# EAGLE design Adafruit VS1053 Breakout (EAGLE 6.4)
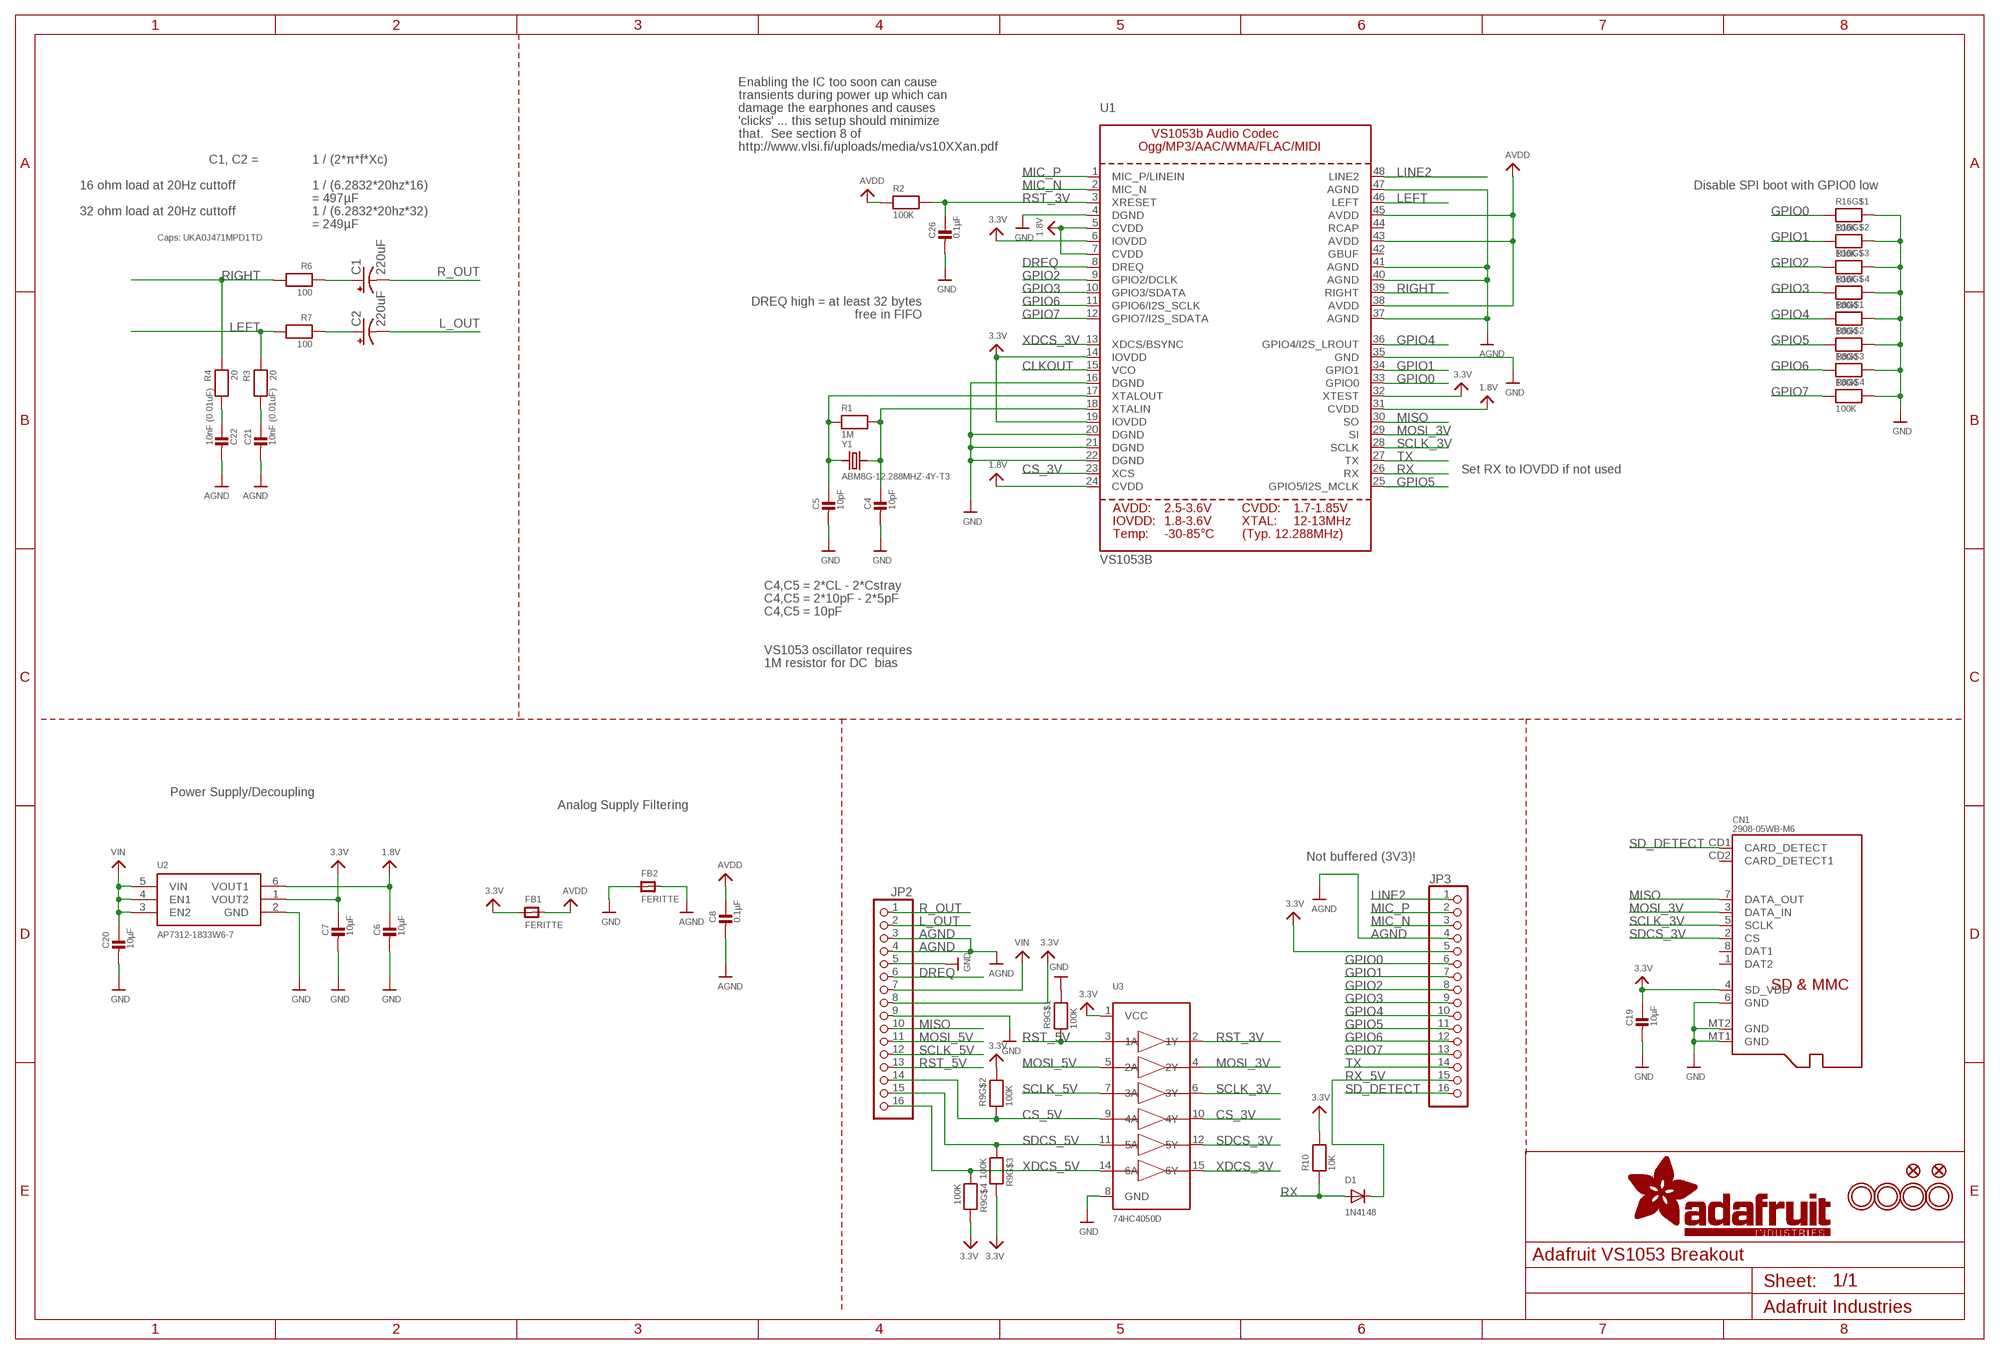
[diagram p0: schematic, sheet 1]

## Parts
C1  220uF  CPOL-USC  [PANASONIC_C]
C2  220uF  CPOL-USC  [PANASONIC_C]
C4  10pF  CAP_CERAMIC_0805MP  [_0805MP]
C5  10pF  CAP_CERAMIC_0805MP  [_0805MP]
C6  10µF  CAP_CERAMIC_0805MP  [_0805MP]
C7  10µF  CAP_CERAMIC_0805MP  [_0805MP]
C8  0.1µF  CAP_CERAMIC_0805MP  [_0805MP]
C19  10µF  CAP_CERAMIC_0805MP  [_0805MP]
C20  10µF  CAP_CERAMIC_0805MP  [_0805MP]
C21  10nF (0.01uF)  CAP_CERAMIC_0805MP  [_0805MP]
C22  10nF (0.01uF)  CAP_CERAMIC_0805MP  [_0805MP]
C26  0.1µF  CAP_CERAMIC_0805MP  [_0805MP]
CN1  2908-05WB-M6  MICROSD  [MICROSD]
D1  1N4148  DIODESOD-323  [SOD-323]
FB1  FERITTE  FERRITE_0805MP  [_0805MP]
FB2  FERITTE  FERRITE_0805MP  [_0805MP]
FID1  FIDUCIAL""  [FIDUCIAL_1MM]
FID2  FIDUCIAL""  [FIDUCIAL_1MM]
JP2  HEADER-1X16ROUND  [1X16_ROUND]
JP3  HEADER-1X16ROUND  [1X16_ROUND]
R1  1M  RESISTOR_0805MP  [_0805MP]
R2  100K  RESISTOR_0805MP  [_0805MP]
R3  20  RESISTOR_0805MP  [_0805MP]
R4  20  RESISTOR_0805MP  [_0805MP]
R6  100  RESISTOR_0805MP  [_0805MP]
R7  100  RESISTOR_0805MP  [_0805MP]
R8  100K  RESISTOR_4PACK  [RESPACK_4X0603]
R9  100K  RESISTOR_4PACK  [RESPACK_4X0603]
R10  10K  RESISTOR0805_NOOUTLINE  [0805-NO]
R16  100K  RESISTOR_4PACK  [RESPACK_4X0603]
U1  VS1053B  [LQFP48]
U2  AP7312-1833W6-7  VREG_SOT23-6_DUALAP7312  [SOT23-6]
U3  74HC4050D  [SOIC16]
U$50  MOUNTINGHOLE3.0THIN  [MOUNTINGHOLE_3.0_PLATEDTHIN]
U$51  MOUNTINGHOLE3.0THIN  [MOUNTINGHOLE_3.0_PLATEDTHIN]
U$52  MOUNTINGHOLE3.0THIN  [MOUNTINGHOLE_3.0_PLATEDTHIN]
U$53  MOUNTINGHOLE3.0THIN  [MOUNTINGHOLE_3.0_PLATEDTHIN]
Y1  ABM8G-12.288MHZ-4Y-T3  CRYSTAL3.2X2.5  [CRYSTAL_3.2X2.5]

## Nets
1.8V: C6.1 U1.5(CVDD) U1.7(CVDD) U1.24(CVDD) U1.31(CVDD) U2.6(VOUT1)
3.3V: C7.1 C19.1 CN1.4(SD_VDD) FB1.1 JP2.8 JP3.5 R9.5 R9.6 R9.7 R10.2 U1.6(IOVDD) U1.14(IOVDD) U1.19(IOVDD) U1.32(XTEST) U2.1(VOUT2) U3.1(VCC)
AGND: C8.2 C21.2 C22.2 FB2.2 JP2.3 JP2.4 JP3.4 U1.37(AGND) U1.40(AGND) U1.41(AGND) U1.47(AGND)
AVDD: C8.1 FB1.2 R2.1 U1.38(AVDD) U1.43(AVDD) U1.45(AVDD)
CLKOUT: U1.15(VCO)
CS_3V: U1.23(XCS) U3.10(4Y)
CS_5V: JP2.14 R9.2 U3.9(4A)
DREQ: JP2.6 U1.8(DREQ)
GND: C4.2 C5.2 C6.2 C7.2 C19.2 C20.2 C26.2 CN1.6(GND) CN1.MT1(GND) CN1.MT2(GND) FB2.1 JP2.5 JP2.9 R8.5 R8.6 R8.7 R8.8 R9.8 R16.5 R16.6 R16.7 R16.8 U1.4(DGND) U1.16(DGND) U1.20(DGND) U1.21(DGND) U1.22(DGND) U1.35(GND) U2.2(GND) U3.8(GND)
GPIO0: JP3.6 R16.1 U1.33(GPIO0)
GPIO1: JP3.7 R16.2 U1.34(GPIO1)
GPIO2: JP3.8 R16.3 U1.9(GPIO2/DCLK)
GPIO3: JP3.9 R16.4 U1.10(GPIO3/SDATA)
GPIO4: JP3.10 R8.1 U1.36(GPIO4/I2S_LROUT)
GPIO5: JP3.11 R8.2 U1.25(GPIO5/I2S_MCLK)
GPIO6: JP3.12 R8.3 U1.11(GPIO6/I2S_SCLK)
GPIO7: JP3.13 R8.4 U1.12(GPIO7/I2S_SDATA)
L_OUT: C2.- JP2.2
LEFT: R3.1 R7.2 U1.46(LEFT)
LEFT_FILTERED: C2.+ R7.1
LINE2: JP3.1 U1.48(LINE2)
MIC_N: JP3.3 U1.2(MIC_N)
MIC_P: JP3.2 U1.1(MIC_P/LINEIN)
MISO: CN1.7(DATA_OUT) JP2.10 U1.30(SO)
MOSI_3V: CN1.3(DATA_IN) U1.29(SI) U3.4(2Y)
MOSI_5V: JP2.11 U3.5(2A)
N$1: C5.1 R1.1 U1.17(XTALOUT) Y1.1
N$2: C4.1 R1.2 U1.18(XTALIN) Y1.2
N$5: C21.1 R3.2
N$6: C22.1 R4.2
R_OUT: C1.- JP2.1
RIGHT: R4.1 R6.2 U1.39(RIGHT)
RIGHT_FILTERED: C1.+ R6.1
RST_3V: C26.1 R2.2 U1.3(XRESET) U3.2(1Y)
RST_5V: JP2.13 R9.1 U3.3(1A)
RX: D1.A R10.1 U1.26(RX)
RX_5V: D1.C JP3.15
SCLK_3V: CN1.5(SCLK) U1.28(SCLK) U3.6(3Y)
SCLK_5V: JP2.12 U3.7(3A)
SD_DETECT: CN1.CD1(CARD_DETECT) JP3.16
SDCS_3V: CN1.2(CS) U3.12(5Y)
SDCS_5V: JP2.15 R9.3 U3.11(5A)
TX: JP3.14 U1.27(TX)
VIN: C20.1 JP2.7 U2.3(EN2) U2.4(EN1) U2.5(VIN)
XDCS_3V: U1.13(XDCS/BSYNC) U3.15(6Y)
XDCS_5V: JP2.16 R9.4 U3.14(6A)
Unconnected: CN1.1(DAT2) CN1.8(DAT1) CN1.CD2(CARD_DETECT1) U1.42(GBUF) U1.44(RCAP)

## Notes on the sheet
- Enabling the IC too soon can cause
- transients during power up which can
- damage the earphones and causes
- 'clicks' ... this setup should minimize
- that.  See section 8 of
- http://www.vlsi.fi/uploads/media/vs10XXan.pdf
- C1, C2 = | 1 / (2*π*f*Xc)
- 16 ohm load at 20Hz cuttoff | 1 / (6.2832*20hz*16) | Disable SPI boot with GPIO0 low
- = 497µF
- 32 ohm load at 20Hz cuttoff | 1 / (6.2832*20hz*32)
- = 249µF
- Caps: UKA0J471MPD1TD
- DREQ high = at least 32 bytes
- free in FIFO
- Set RX to IOVDD if not used
- C4,C5 = 2*CL - 2*Cstray
- C4,C5 = 2*10pF - 2*5pF
- C4,C5 = 10pF
- VS1053 oscillator requires
- 1M resistor for DC  bias
- Power Supply/Decoupling
- Analog Supply Filtering
- Not buffered (3V3)!

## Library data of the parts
C1 C2 = rcl:CPOL-US: POLARIZED CAPACITOR, American symbol
C4-C8 C19-C22 C26 = microbuilder:CAP_CERAMIC: Ceramic Capacitors
CN1 = microbuilder:MICROSD: MicroSD/Transflash Card Holder with SPI pinout 3M: 2908-05WB-MG 4UConnector: 19656 Footprint courtesy: Adafruit Industries
D1 = microbuilder:DIODE: Diode
FB1 FB2 = microbuilder:FERRITE: Ferrite Bead
FID1 FID2 = microbuilder:FIDUCIAL: Fiducial Alignment Points; BOM: EXCLUDE
JP2 JP3 = microbuilder:HEADER-1X16: PIN HEADER
R1-R4 R6 R7 R10 = microbuilder:RESISTOR: Resistors
R8 R9 R16 = microbuilder:RESISTOR_4PACK: Resistor Packs (4 resistors) 4 x 0603 10K 1/16W - Digikey: YC164J-10KCT-ND
U1 = microbuilder:VS1053B: VS1053b Audio Codec - Ogg Vorbis/MP3/AAC/WMA/FLAC/MIDI
U2 = microbuilder:VREG_SOT23-6_DUAL: Dual Output SOT23-6 Linear Regulators Diodes Inc. AP7312 - Dual 150mA LDO Linear Regulator 0.2V dropout, 150mA output, 2-6V Input AP7312-1833W6-7 - 1.8V/3.3V SOT23-6 (Digikey: AP7312-1833W6-7DICT-ND) MIC5320 - Dual 150mA ULDO Linear Regulator Ultra-low 35mV dropout at 150mA, 2.3-5.5V Input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
U3 = microbuilder:74HC4050D: 6-channel level shifter 74HC4050D - 2V-6V Supply SOIC16 Digikey: 74HC4050D,653-ND Mouser: 771-74HC4050D-T TSSOP16 Digikey: 296-9215-1-ND Mouser:
U$50-U$53 = microbuilder:MOUNTINGHOLE: Mounting Hole; BOM: EXCLUDE
Y1 = microbuilder:CRYSTAL: Crystals

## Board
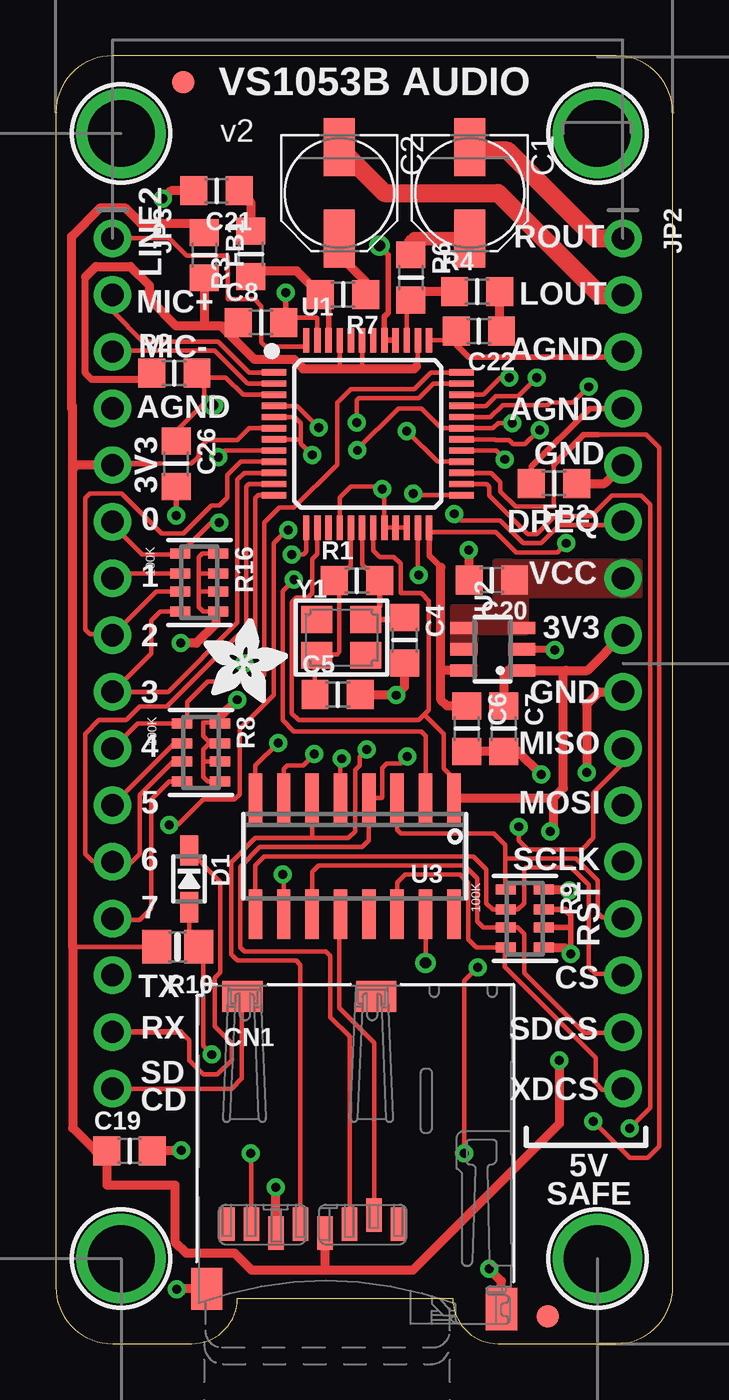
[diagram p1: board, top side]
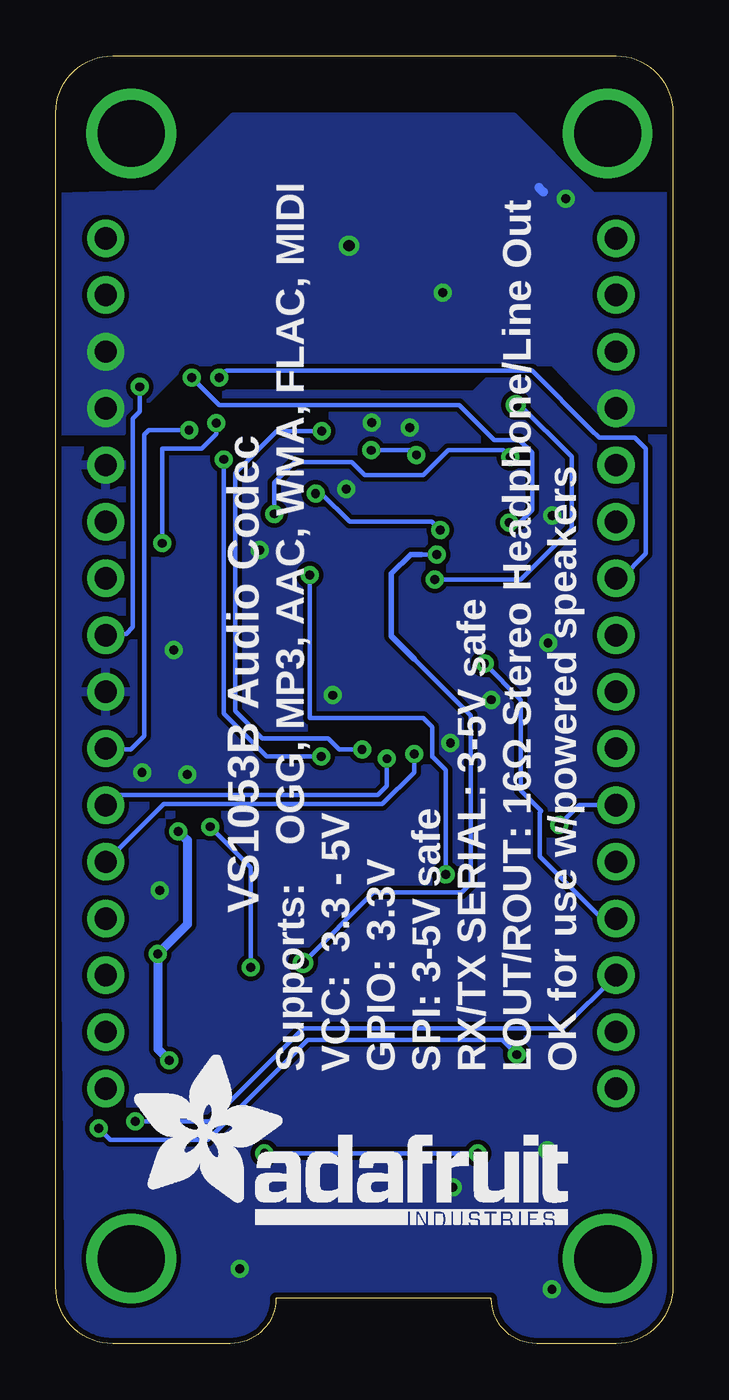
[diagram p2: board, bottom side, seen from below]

Size 27.64 x 57.71 mm. Coordinates in mm from the lower left corner, seen from the top.
Outline: 19.81,0 25.09,0 arc90 27.64,2.54 27.64,55.17 arc90 25.09,57.71 2.54,57.71 arc90 0,55.17 0,2.54 arc90 2.54,0 6.1,0 arc90 8.13,2.03 17.78,2.03 arc90 19.81,0
Copper layers (1*16): Top 0.035mm / dielectric 1.5mm / Bottom 0.035mm
Design rules "adafruit *": minimum track width 8mil, minimum drill 15.5mil, track to track 8mil, track to pad 8mil, pad to pad 8mil, via to via 8mil, smd to smd 8mil, copper to edge 10mil, drill to drill 8mil, minimum pad ring 10mil, minimum via ring 8mil, stop-mask expansion 4mil, vias tented up to drill 20mil, thermal gap 10mil

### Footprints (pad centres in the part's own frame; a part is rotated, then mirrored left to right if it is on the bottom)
PANASONIC_C = smd 2.6 x 1.4: + 2.05,0; - -2.05,0
_0805MP = smd 1.2 x 1.3: 1 -1.016,0; 2 1.016,0
MICROSD = smd 0.7 x 1.5: 1 9,-10.64; 2 7.9,-10.24; 3 6.8,-10.64; 4 5.7,-11.04; 5 4.6,-10.64; 6 3.5,-11.04; 7 2.4,-10.64; 8 1.3,-10.64 | smd 1.8 x 1.4: CD1 2,-0.44; CD2 8,-0.44 | smd 1.4 x 1.9: MT1 0.4,-13.54; MT2 13.6,-14.44
SOD-323 = smd 1.35 x 0.8: A 1.27,0; C -1.27,0
FIDUCIAL_1MM = smd 1 x 1: 1 0,0
1X16_ROUND = drill 1 pad 1.676: 1 -19.05,0; 2 -16.51,0; 3 -13.97,0; 4 -11.43,0; 5 -8.89,0; 6 -6.35,0; 7 -3.81,0; 8 -1.27,0; 9 1.27,0; 10 3.81,0; 11 6.35,0; 12 8.89,0; 13 11.43,0; 14 13.97,0; 15 16.51,0; 16 19.05,0
RESPACK_4X0603 = smd 0.45 x 0.9: 1 -1.3,-0.85; 2 -0.4,-0.85; 3 0.4,-0.85; 4 1.3,-0.85; 5 1.3,0.85; 6 0.4,0.85; 7 -0.4,0.85; 8 -1.3,0.85
0805-NO = smd 1.3 x 1.5: 1 -0.95,0; 2 0.95,0
LQFP48 = smd 1.1 x 0.285: 1 -4.2,2.75; 2 -4.2,2.25; 3 -4.2,1.75; 4 -4.2,1.25; 5 -4.2,0.75; 6 -4.2,0.25; 7 -4.2,-0.25; 8 -4.2,-0.75; 9 -4.2,-1.25; 10 -4.2,-1.75; 11 -4.2,-2.25; 12 -4.2,-2.75; 25 4.2,-2.75; 26 4.2,-2.25; 27 4.2,-1.75; 28 4.2,-1.25; 29 4.2,-0.75; 30 4.2,-0.25; 31 4.2,0.25; 32 4.2,0.75; 33 4.2,1.25; 34 4.2,1.75; 35 4.2,2.25; 36 4.2,2.75 | smd 0.285 x 1.1: 13 -2.75,-4.2; 14 -2.25,-4.2; 15 -1.75,-4.2; 16 -1.25,-4.2; 17 -0.75,-4.2; 18 -0.25,-4.2; 19 0.25,-4.2; 20 0.75,-4.2; 21 1.25,-4.2; 22 1.75,-4.2; 23 2.25,-4.2; 24 2.75,-4.2; 37 2.75,4.2; 38 2.25,4.2; 39 1.75,4.2; 40 1.25,4.2; 41 0.75,4.2; 42 0.25,4.2; 43 -0.25,4.2; 44 -0.75,4.2; 45 -1.25,4.2; 46 -1.75,4.2; 47 -2.25,4.2 | smd 0.28 x 1.1: 48 -2.75,4.2
SOT23-6 = smd 0.55 x 1.2: 1 -0.95,-1.3; 2 0,-1.3; 3 0.95,-1.3; 4 0.95,1.3; 5 0,1.3; 6 -0.95,1.3
SOIC16 = smd 0.6 x 2.2: 1 -4.445,-2.6; 2 -3.175,-2.6; 3 -1.905,-2.6; 4 -0.635,-2.6; 5 0.635,-2.6; 6 1.905,-2.6; 7 3.175,-2.6; 8 4.445,-2.6; 9 4.445,2.6; 10 3.175,2.6; 11 1.905,2.6; 12 0.635,2.6; 13 -0.635,2.6; 14 -1.905,2.6; 15 -3.175,2.6; 16 -4.445,2.6
MOUNTINGHOLE_3.0_PLATEDTHIN = drill 3 pad 3.6: P$1 0,0
CRYSTAL_3.2X2.5 = smd 1.4 x 1.2: 1 -1.1,-0.8; 2 1.1,0.8; GND1 -1.1,0.8; GND2 1.1,-0.8

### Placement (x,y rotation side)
C1  18.54,51.56 270 top
C2  12.7,51.56 270 top
C4  15.62,31.52 270 top
C5  12.62,29.08 0 top
C6  18.41,27.56 270 top
C7  20.07,27.56 270 top
C8  9.19,45.76 0 top
C19  3.3,8.64 0 top
C20  19.53,34.21 180 top
C21  7.2,51.66 180 top
C22  18.95,45.37 180 top
C26  5.38,39.43 270 top
CN1  6.36,16 0 top
D1  5.97,20.83 270 top
FB1  6.66,48.77 270 top
FB2  22.32,38.55 180 top
FID1  5.71,56.52 0 top
FID2  22.04,1.22 0 top
JP2  25.4,30.48 270 top
JP3  2.54,30.48 270 top
R1  13.49,34.19 0 top
R2  5.31,43.49 0 top
R3  8.73,48.83 90 top
R4  18.87,47.14 0 top
R6  15.91,47.77 270 top
R7  12.86,47.01 180 top
R8  6.5,26.49 270 top
R9  21.01,19.05 270 top
R10  5.46,17.78 180 top
R16  6.43,34.11 270 top
U1  13.97,40.77 0 top
U2  19.57,31.12 90 top
U3  13.39,21.84 180 top
U$31  [ADAFRUIT_3.5MM]  6.6,28.7 0 top
U$50  2.92,3.81 0 top
U$51  24.26,3.81 0 top
U$52  24.26,54.23 0 top
U$53  2.92,54.23 0 top
U$55  [ADAFRUIT_TEXT_20MM]  24.28,5.33 0 bottom
Y1  12.79,31.64 0 top

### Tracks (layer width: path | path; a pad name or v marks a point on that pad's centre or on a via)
1.8V  (via drill 0.4)
  Top 0.203: U1.5 10.71,41.52 10.97,41.25 10.97,40.54 | 10.97,40.54 10.97,40.34 v11.48,39.83 | U1.7 10.95,40.52 10.97,40.54 | v22.86,35.87 22.45,35.46 20.62,35.46 19.71,36.37 16.76,36.37 16.72,36.42 U1.24 | v13.51,40.03 13.46,40.03 15.34,41.91 16.38,41.91 17.27,41.02 U1.31 | v20.45,41.25 19.82,41.25 19.81,41.25 19.58,41.02 U1.31 | U1.31
  Top 0.254: U1.24 16.72,35.33 17.25,34.8
  Top 0.406: C6.1 17.53,28.57 17.25,28.85 17.25,30.23 | 17.25,30.23 17.25,34.8 | U2.6 17.3,30.17 17.25,30.23
  Bottom 0.203: v13.51,40.03 11.68,40.03 v11.48,39.83 | v22.86,35.87 22.86,40.1 21.1,40.1 20.45,40.75 v20.45,41.25
3.3V  (via drill 0.4)
  Top 0.203: 16.51,28.19 16.71,28.4 16.71,33.27 16.36,33.63 15.44,33.63 15.44,34.95 15.14,35.26 14.5,35.26 14.22,35.54 U1.19 | 16.51,28.19 16.26,27.94 10.87,27.94 10.57,28.25 10.57,33.22 10.77,33.43 11.28,33.43 11.48,33.63 11.48,35.15 11.72,35.39 U1.14 | U3.1 17.78,24.5 17.78,25.38 17.37,25.78 17.37,27.33 16.51,28.19 | v23.88,42.88 23.16,42.16 22.15,42.16 22.04,42.06 20.01,42.06 19.47,41.52 U1.32 | U1.6 8.66,41.02 8.13,40.49 6.79,40.49 6.4,40.1 6.4,39.76 | 6.4,39.76 6.4,39.7 | 4.42,39.43 6.07,39.43 6.4,39.76 | R10.2 0.75,17.78
  Top 0.254: R9.7 22.82,19.45 23.06,19.2 23.06,18.59 | 23.06,18.59 v23.06,17.48 | R9.6 23.01,18.65 23.06,18.59 | 4.42,39.43 2.6,39.43 JP3.5
  Top 0.406: 0.71,41.91 0.71,42.04 | 0.71,42.04 0.71,49.61 2,50.9 3.1,50.9 3.8,50.2 6.5,50.2 6.5,49.95 FB1.1 | C7.1 20.07,29.97 20.26,30.17 U2.1 22.86,30.17 | 22.86,30.17 23.82,30.17 JP2.8 | U3.1 22.29,24.44 | 22.29,24.44 22.73,24.89 22.73,30.04 22.86,30.17 | CN1.4 12.06,3.38 11.99,3.3 | R9.5 22.79,17.75 v23.06,17.48 | v22.55,12.7 22.55,9.86 16,3.3 11.99,3.3 | 11.99,3.3 8.76,3.3 8,4.06 5.84,4.06 5.33,4.57 5.33,7.11 2.29,7.11 C19.1 1.78,8.64 0.75,9.67 0.75,17.78 0.75,39.2 | 22.29,24.44 22.29,23.1 v22.15,22.96 | 0.75,39.2 0.75,42 0.71,42.04 | JP3.5 0.92,39.37 0.75,39.2
  Bottom 0.203: v23.88,42.88 23.88,41.76 24.18,41.45 24.18,32.11 24.49,31.8 25.35,31.8 JP2.8
  Bottom 0.406: v22.55,12.7 23.06,13.21 v23.06,17.48 21.74,18.8 21.74,22.55 v22.15,22.96
AGND  (via drill 0.4, 0.5)
  Top 0.203: U1.37 17.8,44.97 17.94,44.83 | U1.47 11.72,45.94 11.68,45.97 10.42,45.97 C8.2
  Top 0.254: FB2.2 21.3,39.3 23.91,41.91 JP2.4 | C22.2 17.94,44.83 17.94,44.76 18.5,44.2 25.15,44.2 JP2.3 | U1.40 U1.41 14.72,46.02 14.9,46.2 14.9,48.8 v14.5,49.2 | 10.3,45.85 v10.3,47.1 | 10.64,46.2 10.56,46.12 | 10.56,46.12 10.3,45.85 | 10.54,46.12 10.56,46.12 | 10.3,45.85 C8.2
  Top 0.406: C21.2 5.16,51.66 v4.8,51.3
  Bottom 0.254: v14.5,49.2 14.6,49.2 14.7,49.3
  Bottom 0.406: 6,51.8 5.8,51.6
  pour Bottom (no thermals): 0,41.18 2.77,41.18 5.38,43.89 21.84,43.89 24.59,41.15 24.59,40.8 26.11,40.8 27.61,40.78 27.61,51.49 23.16,51.61 19.71,55.07 7.11,55.07 3.56,51.51 0,51.51
AVDD
  Top 0.203: U1.38 16.22,43.85 16.15,43.79 | 13.82,43.69 13.72,43.79 U1.43 | U1.45 12.72,43.71 12.7,43.69 | 3.71,43.2 4.09,43.59 | 8.01,45.6 8.18,45.6 C8.1
  Top 0.254: 4.09,43.59 4.19,43.59 R2.1 | 7.71,45.6 8.01,45.6
  Top 0.305: 3.71,43.2 1.6,43.2 1.32,43.48 1.32,47.79
  Top 0.406: 16.15,43.79 16.05,43.69 13.82,43.69 12.7,43.69 11.07,43.69 10.66,44.1 8.9,44.1 7.4,45.6 | 1.32,47.79 1.79,48.26 3.34,48.26 4.2,47.4 4.2,46.8 5.4,45.6 6.7,45.6 | 7.4,45.6 6.7,45.6 | 7.4,45.6 7.71,45.6 | FB1.2 6.66,45.64 6.7,45.6
CS_3V  (via drill 0.4)
  Top 0.203: U3.10 10.21,20.98 v10.16,21.03 | U1.23 16.22,34.48 v16.26,34.44
  Bottom 0.203: v10.16,21.03 10.16,25.7 10.74,26.29 10.77,26.29 10.77,27.64 11.18,28.04 16.26,28.04 v16.26,34.44
CS_5V
  Top 0.203: U3.9 8.94,21.44 9.35,21.84 18.69,21.84 19.28,21.26 19.28,19.74 19.56,19.45 R9.2 20.7,19.45 20.98,19.74 20.98,21.26 21.06,21.34 23.09,21.34 23.88,20.55 23.88,16.87 24.18,16.56 25.35,16.56 JP2.14
DREQ  (via drill 0.4)
  Top 0.203: 25.35,36.88 JP2.6 25.25,36.68 22.55,36.68 21.74,35.87 20.93,35.87 19.91,36.88 18.16,36.88 v17.86,37.19 | U1.8 7.58,40.02 v7.29,39.73
  Bottom 0.203: v7.29,39.73 7.59,40.03 10.06,40.03 11.18,38.91 13.79,38.91 14.38,39.5 16.94,39.5 17.86,38.58 v17.86,37.19 17.88,37.19
GND  (via drill 0.4)
  Top 0.203: R8.5 6.81,25.19 6.6,25.4 6.6,26.11 | 6.6,26.11 6.6,26.62 6.88,26.89 R8.7 6.94,26.89 6.6,27.23 6.6,27.84 7.31,27.84 R8.8 | R8.6 6.62,26.09 6.6,26.11 | R16.8 6.56,35.41 6.4,35.26 6.4,34.54 | 6.4,34.54 6.4,33.73 | 6.4,33.73 6.4,33.02 6.6,32.82 7.17,32.82 | R16.6 6.42,33.71 6.4,33.73 | R16.7 6.43,34.51 6.4,34.54 | U1.16 12.72,37.92 13.21,38.41 14.53,38.41 v14.63,38.3 14.72,38.21 U1.20 U1.21 U1.22 | U1.35 16.91,43.02 16.26,42.37 13.56,42.37 13.49,42.29 v13.49,41.27 | U1.4 10.81,42.02 v11.79,41.05 | U3.8 8.94,25.91 v9.96,26.92 | 7.37,28.1 7.38,28.09
  Top 0.254: C26.2 5.38,37.12 v5.4,37.1
  Top 0.305: U2.2 22.32,31.12 v22.35,31.09
  Top 0.406: v8.13,28.85 7.37,28.1 7.37,27.81 R8.8 | v5.59,31.39 6.3,31.39 7.18,32.27 7.18,32.71 R16.5 7.18,32.81 7.17,32.82 | C20.2 18.52,35.53 v18.49,35.56 | v23.77,25.6 23.77,28.65 24.33,29.21 JP2.9 | C6.2 C7.2 20.7,26.54 v21.74,25.5 | C5.2 15.21,29.08 v15.24,29.06 15.62,29.44 C4.2 | R9.8 22.96,20.35 v22.99,20.32 | CN1.6 v9.86,7.01 | CN1.MT1 5.43,2.46 v5.41,2.44 | CN1.MT2 19.96,2.8 v19.41,3.35 | v5.61,8.66 5.59,8.64 C19.2 | FB2.1 24.58,38.55 JP2.5
  pour Bottom: 0,40.57 2.77,40.47 5.8,43.2 8.1,43.3 8.9,42.5 21.54,42.57 23.27,40.84 23.27,39.99 27.43,39.99 27.03,0 0,0
GPIO0  (via drill 0.4)
  Top 0.203: JP3.6 2.54,36.68 3.86,35.36 5.62,35.36 5.62,35.37 R16.1 6.95,36.79 7.05,36.79 | v21.54,43.28 20.72,42.47 19.71,42.47 19.26,42.02 U1.33
  Top 0.254: 7.05,36.79 v7.32,36.79
  Bottom 0.203: v21.54,43.28 20.32,42.06 9.56,42.06 8,40.5 6.87,40.5 6.3,39.93 6.3,37.35 6.86,36.79
  Bottom 0.254: 6.86,36.79 | 6.86,36.79 v7.32,36.79
GPIO1  (via drill 0.4)
  Top 0.203: 2.56,34.31 JP3.7 2.76,34.51 R16.2 | U1.34 19.15,42.52 19.91,43.28 v20.32,43.28
  Bottom 0.203: 20.22,43.18 v20.32,43.28 20,43.6 6.3,43.6 3.66,40.96 3.3,40.6 1.7,40.6 1.2,40.1 1.2,35.4 2.31,34.29 JP3.7
GPIO2
  Top 0.203: R16.3 4.5,33.71 JP3.8 2.49,31.8 1.52,31.8 1.32,32 1.32,37.9 1.52,38.1 2.95,38.1 4.75,36.3 5.7,36.3 6.96,37.55 7.32,37.55 7.67,37.91 7.67,38.91 8.28,39.52 U1.9
GPIO3
  Top 0.203: U1.10 8.44,39.02 8.13,38.71 8.13,32.31 5.03,29.21 JP3.9 4.27,30.94 4.27,32.41 4.67,32.81 R16.4
  Bottom 0.203: 2.59,29.16 JP3.9
GPIO4
  Top 0.203: JP3.10 3.66,27.79 R8.1 5.89,28.03 5.89,28.75 6.81,29.67 9.04,29.67 9.35,29.97 9.35,36.8 10.01,37.47 10.67,37.47 12.6,39.4 12.6,42.16 13.21,42.77 16.05,42.77 16.8,43.52 U1.36
GPIO5  (via drill 0.4)
  Top 0.203: R8.2 5.3,26.89 JP3.11 | v5.08,23.24 5.46,23.24 6.6,24.38 8,24.38 8.23,24.61 8.23,27.53 9.75,29.06 9.75,35.87 10.34,36.45 v10.41,36.45 | v16,38.1 16.09,38.02 U1.25
  Bottom 0.203: JP3.11 4.19,24.13 v5.08,23.24 | v10.41,36.45 10.79,36.83 14.48,36.83 15.75,38.1 v16,38.1
GPIO6
  Top 0.203: R8.3 5.26,26.09 3.76,24.59 3.76,21.95 3.35,21.54 2.59,21.54 JP3.12 2.49,21.64 1.63,21.64 1.32,21.95 1.32,27.33 1.93,27.94 3.15,27.94 3.76,28.55 4.98,28.55 8.53,32.11 8.53,38.41 8.65,38.52 U1.11
GPIO7  (via drill 0.4)
  Top 0.203: JP3.13 2.59,19 3.76,19 4.27,19.51 4.27,24.38 5.08,25.19 R8.4 | U1.12 9.06,38.02 8.94,37.9 8.94,30.99 v8.43,30.48
  Bottom 0.203: v8.43,30.48 6.81,28.85 6.81,24.79 5.89,23.88 5.97,23.8 5.97,21.84 3.17,19.05 JP3.13
L_OUT
  Top 0.813: C2.- 12.7,53.59 14.73,51.56 19.81,51.56 24.38,46.99 JP2.2
LEFT
  Top 0.254: U1.46 12.22,46.84 12.05,47.01 R7.2
  Top 0.406: R3.1 8.97,48.06 10.8,48.06 R7.2
LEFT_FILTERED
  Top 0.406: R7.1 13.88,47.59 12.7,48.77 C2.+
LINE2
  Top 0.203: JP3.1 5.07,49.53 5.85,48.75 7.65,48.75 7.7,48.7 7.7,46.8 8.9,46.8 9.2,46.5 9.2,44.87 9.4,44.67 11.22,44.67 U1.48
MIC_N
  Top 0.203: U1.2 8.6,43.02 7.12,44.5 2.6,44.5 arc60 JP3.3
MIC_P
  Top 0.203: U1.1 8.67,43.52 7.28,44.9 3.9,44.9 2.54,46.26 JP3.2
MISO  (via drill 0.4)
  Top 0.203: CN1.7 8.76,8.51 v8.74,8.53 | v18.29,8.53 18.29,16.26 v18.9,16.87 | v20.73,23.16 20.73,22.55 21.13,22.15 23.57,22.15 24.08,22.66 24.08,24.69 25.3,25.91 25.3,26.57 JP2.10 | U1.30 19.69,40.52 19.71,40.5 20.3,40.5 20.5,40.3 21,40.3 21.65,40.95 v21.67,40.95
  Bottom 0.203: JP2.10 25.35,26.62 24.28,26.62 23.67,27.23 23.67,40.74 23.47,40.95 v21.67,40.95 | v8.74,8.53 v18.29,8.53 | v18.9,16.87 18.9,21.34 v20.73,23.16
MOSI_3V  (via drill 0.4)
  Top 0.203: CN1.3 13.16,13.77 12.29,14.63 12.29,17.37 12.09,17.58 8.43,17.58 8.26,17.75 8.26,21.36 9.14,22.25 13.72,22.25 14.02,22.55 U3.4 14.59,24.44 14.63,24.49 14.63,25.81 14.83,26.01 15.44,26.01 v15.75,26.31 | v20.11,39.63 19.72,40.02 U1.29
  Bottom 0.203: v15.75,26.31 18.19,26.31 20.11,28.24 v20.11,39.63
MOSI_5V  (via drill 0.4)
  Top 0.203: U3.5 12.75,26.16 v12.8,26.21
  Bottom 0.203: v12.8,26.21 12.8,24.99 13.21,24.59 24.94,24.59 JP2.11
N$1
  Top 0.203: R1.1 12.24,34.19 | 11.63,29.1 C5.1 11.61,30.76 Y1.1 11.73,30.89 12.6,30.89 12.7,30.99 12.7,33.83 12.47,34.06 R1.1 | U1.17 13.22,34.86 12.55,34.19 R1.1
N$2
  Top 0.203: U1.18 13.72,34.92 14.45,34.19 R1.2
  Top 0.254: R1.2 14.5,33.06 Y1.2 15.62,32.44 C4.1
N$5
  Top 0.406: C21.1 8.73,51.14 R3.2
N$6
  Top 0.406: C22.1 19.89,45.37 R4.2
R_OUT
  Top 0.813: JP2.1 24.17,49.53 20.25,53.45 18.7,53.45 C1.-
RIGHT
  Top 0.203: 15.71,46.76 15.71,46.95 15.9,47.14 | U1.39 15.72,46.57 R6.2
  Top 0.254: 15.71,46.76 R6.2
  Top 0.406: R4.1 15.9,47.14 15.71,47.14
RIGHT_FILTERED
  Top 0.61: C1.+ 16.07,49.51 15.91,49.35 R6.1
RST_3V  (via drill 0.4, 0.5)
  Top 0.203: U1.3 8.38,42.52 7.62,43.28 6.53,43.28 R2.2 6.43,43.39 6.43,43.08 6.66,42.85 6.66,42.49 6.99,42.16 6.99,42.11 v7.04,42.06 6.56,42.06 5.38,40.88 C26.1 | U3.2 16.56,27.23 16.36,27.43 10.67,27.43 10.16,27.94 10.16,33.73 v10.67,34.24
  Bottom 0.203: v10.67,34.24 6.81,34.24 4.53,36.51 4.53,39.75 6.84,42.06 v7.04,42.06
RST_5V
  Top 0.203: U3.3 15.29,23.01 15.44,22.86 19.61,22.86 20.13,22.34 20.13,21.74 | 20.13,21.74 23.29,21.74 24.28,20.75 24.28,19.3 24.49,19.1 25.35,19.1 JP2.13 | 20.13,21.74 20.13,20.32 R9.1
RX  (via drill 0.4)
  Top 0.203: U1.26 19.29,38.52 19.41,38.4 19.41,37.99 21.13,36.27 21.54,36.27 22.35,37.08 23.98,37.08 24.89,38 26.21,38 26.62,37.59 26.62,10.57 v25.7,9.65 | v6.99,12.95 6.6,13.34 6.6,17.59 R10.1 5.97,18.22 D1.A
  Bottom 0.203: v25.7,9.65 25.2,9.14 20.83,9.14 16.36,13.61 7.64,13.61 v6.99,12.95
RX_5V
  Top 0.203: 5.59,13.97 5.97,13.59 5.97,12.7 6.6,12.06 7.24,12.06 7.87,12.7 7.87,13.46 7.11,14.22 7.11,16.38 7.37,16.64 7.37,20.7 D1.C
  Top 0.254: JP3.15 5.59,13.97
SCLK_3V  (via drill 0.4)
  Top 0.203: CN1.5 10.96,16.98 10.77,17.17 8.13,17.17 7.85,17.45 7.85,21.57 8.94,22.66 11.48,22.66 | 11.48,22.66 13.11,22.66 13.41,22.96 13.41,25.7 13.61,25.91 13.61,26.31 v13.92,26.62 | 11.48,22.66 U3.6 | U1.28 17.1,39.52 v15.72,40.89
  Bottom 0.203: v15.72,40.89 17.73,40.89 19.61,39.01 19.61,28.35 18.39,27.13 15.44,27.13 14.94,26.62 v13.92,26.62
SCLK_5V  (via drill 0.4)
  Top 0.203: U3.7 10.21,25.76 10.36,25.91 11.07,25.91 v11.58,26.42
  Bottom 0.203: v11.58,26.42 11.58,25.6 13.01,24.18 22.81,24.18 JP2.12
SD_DETECT
  Top 0.203: JP3.16 7.87,11.43 8.33,11.89 8.33,15.54 CN1.CD1
SDCS_3V
  Top 0.203: CN1.2 14.26,13.48 12.7,15.04 12.7,19.19 U3.12
SDCS_5V
  Top 0.203: U3.11 11.48,21.13 11.79,21.44 18.29,21.44 18.87,20.85 18.87,18.92 19.14,18.65 R9.3 20.7,18.65 20.98,18.36 20.98,16.61 23.67,13.92 25.35,13.92 JP2.15
TX  (via drill 0.4)
  Top 0.203: U1.27 19.5,39.02 19.91,38.61 19.91,38.19 20.6,37.5 22.3,37.5 22.3,39.4 | v24.08,9.96 25.7,8.33 26.52,8.33 27.03,8.84 27.03,40.16 26.44,40.74 24.29,40.74
  Top 0.254: 22.3,39.4 23.64,40.74 24.29,40.74
  Bottom 0.203: v24.08,9.96 20.73,9.96 16.56,14.12 4.93,14.12 JP3.14
VIN
  pour Top (no thermals): 17.78,30.99 18.8,30.99 18.8,31.88 21.08,31.88 21.08,33.53 26.16,33.53 26.16,35.05 19.68,35.05 19.68,33.02 17.78,33.02
XDCS_3V  (via drill 0.4, 0.5)
  Top 0.203: v16.56,17.07 U3.15 | U1.13 11.22,35.5 11.07,35.36 v10.57,35.36
  Bottom 0.203: 11.58,30.68 9.04,28.14 9.04,20.62 9.45,20.22 13.41,20.22 v16.56,17.07 | 11.27,35.36 v10.57,35.36
  Bottom 0.254: 11.58,30.68 12.6,31.7 12.6,34.5 11.74,35.36 11.27,35.36
XDCS_5V
  Top 0.203: JP2.16 25.35,11.38 24.49,11.38 24.18,11.68 24.18,12.8 20.1,16.88 20.1,17.7 R9.4 18.83,17.75 18.47,18.11 18.47,20.65 18.09,21.03 15.65,21.03 15.29,20.68 U3.14

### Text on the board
tPlace: VS1053B AUDIO | v2 | ROUT | LINE2 | LOUT | MIC+ | AGND | MIC- | AGND | AGND | GND | 3V3 | DREQ | 0 | VCC | 1 | 3V3 | 2 | GND | 3 | MISO | 4 | MOSI | 5 | SCLK | 6 | 7 | RST | CS | TX | SDCS | RX | SD | XDCS | CD | 5V | SAFE
bPlace: OGG, MP3, AAC, WMA, FLAC, MIDI | VS1053B Audio Codec | 3.3V | 3.3 - 5V | OK for use w/powered speakers | LOUT/ROUT: 16Ω Stereo Headphone/Line Out | RX/TX SERIAL: 3-5V safe | SPI: 3-5V safe | GPIO: | VCC: | Supports:
